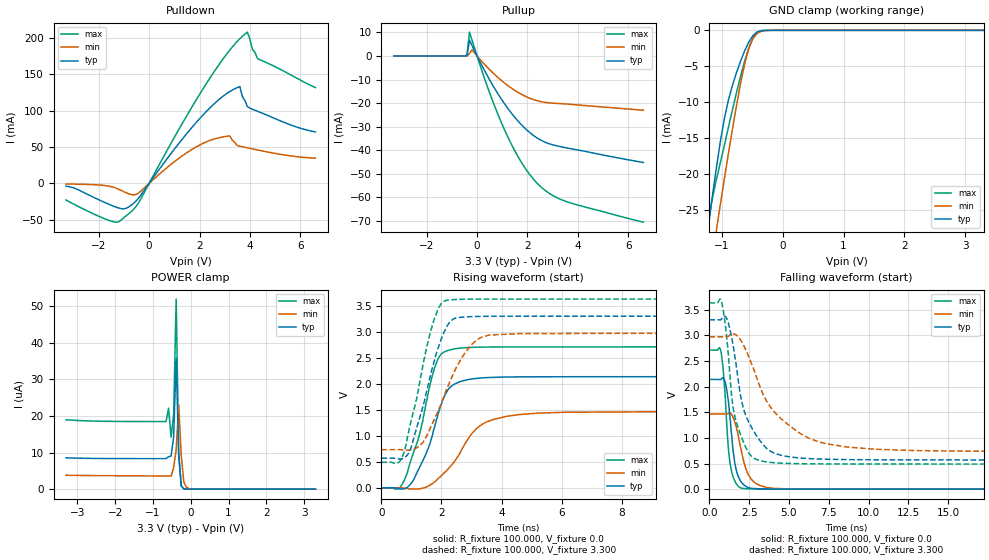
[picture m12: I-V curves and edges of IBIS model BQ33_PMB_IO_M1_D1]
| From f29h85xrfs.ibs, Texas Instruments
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|   Model BQ33_PMB_IO_M1_D1
[Model]   BQ33_PMB_IO_M1_D1
Model_type   I/O
Polarity   Non-Inverting
Enable   Active-Low
Vinl =   0.800V
Vinh =   1.350V
Vmeas =  1.650V
Cref =   100.000pF
Vref =   0.0V
|   typ   min   max
C_comp   1.646pF   1.624pF   1.798pF
[Model Spec]
Vinh   1.350V   1.350V   1.350V
Vinl   0.800V   0.800V   0.800V
[Temperature Range]   30   155   -40
[Voltage Range]   3.300V   2.970V   3.630V
[Pullup Reference]   3.300V   2.970V   3.630V
[Pulldown Reference]   0.0V   0.0V   0.0V
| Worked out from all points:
|   slope of the pulldown table from 0 to 0.495 V, typ, clamps not added: 20.8 ohm
|   slope of the pullup table from 0 to 0.495 V, typ, clamps not added: 49.3 ohm
|   GND clamp passes 1 mA (typ) near -0.51 V on its own axis
|   rising waveform, R_fixture 100.000, V_fixture 0.0: 20-80 % time 762ps typ, 1.14ns min, 712ps max; typ from 0 V to 2.14 V
|   rising waveform, R_fixture 100.000, V_fixture 3.300: 20-80 % time 773ps typ, 1.05ns min, 715ps max; typ from 0.57 V to 3.3 V
|   falling waveform, R_fixture 100.000, V_fixture 0.0: 20-80 % time 455ps typ, 712ps min, 376ps max; typ from 2.14 V to 0 V
|   falling waveform, R_fixture 100.000, V_fixture 3.300: 20-80 % time 1.3ns typ, 2.73ns min, 816ps max; typ from 3.3 V to 0.57 V
[Pulldown]
|Voltage   I(typ)   I(min)   I(max)
-3.3V     -3.922mA   -903.4uA   -22.93mA
-1.4V     -31.61mA   -5.56mA    -53.04mA
-700mV    -29.75mA   -15.51mA   -38.53mA
-400mV    -19.4mA    -12.71mA   -25.68mA
1.5V      68.79mA    42.37mA    93.49mA
2.8V      116.3mA    62.99mA    164.9mA
3.2V      126.4mA    65.38mA    183.5mA
3.6V      133.3mA    51.09mA    199.2mA
3.9V      105.6mA    48.92mA    208.3mA
4.1V      102mA      47.47mA    184.6mA
4.3V      99.3mA     46.01mA    171.8mA
6.6V      70.82mA    34.61mA    131.9mA
[Pullup]
|Voltage   I(typ)   I(min)   I(max)
-3.3V     -1.721nA   13.88nA    1.362nA
-500mV    17.31nA    18.01nA    59.06nA
-400mV    178uA      374.8nA    408.1uA
-300mV    6.695mA    1.073mA    10.14mA
-200mV    4.421mA    2.585mA    6.742mA
400mV     -8.225mA   -4.706mA   -12.71mA
1V        -18.86mA   -10.69mA   -29.15mA
1.7V      -28.49mA   -15.89mA   -44.05mA
2.3V      -34.18mA   -18.71mA   -53.02mA
2.8V      -37mA      -19.82mA   -57.81mA
3.5V      -38.88mA   -20.34mA   -61.59mA
6.6V      -45.18mA   -23.01mA   -70.51mA
[GND_clamp]
|Voltage   I(typ)   I(min)   I(max)
-3.3V     -172.4mA   -156.6mA   -199.3mA
-1.223V   -27.66mA   -35.43mA   -26.88mA
-1.156V   -23.42mA   -31.69mA   -23.55mA
-1.089V   -19.35mA   -27.98mA   -20.9mA
-1.022V   -15.58mA   -24.31mA   -18.47mA
-955mV    -12.3mA    -20.69mA   -16.02mA
-821mV    -7.634mA   -13.71mA   -11.02mA
-620mV    -2.823mA   -4.633mA   -4.248mA
-553mV    -1.627mA   -2.509mA   -2.447mA
-419mV    -233.9uA   -453.9uA   -290.2uA
-218mV    -985nA     -9.253uA   -449.5nA
3.3V      0A         0A         0A
[POWER_clamp]
|Voltage   I(typ)   I(min)   I(max)
-3.3V     8.55uA     3.797uA    18.96uA
-653mV    8.339uA    3.596uA    18.47uA
-586mV    8.872uA    3.591uA    22.11uA
-519mV    9.031uA    3.588uA    14.17uA
-452mV    14.26uA    5.833uA    20.33uA
-385mV    35.62uA    10.82uA    51.91uA
-318mV    9.151uA    22.94uA    10.03uA
-251mV    942nA      9.217uA    856.3nA
-184mV    84.85nA    2.059uA    62.73nA
-117mV    8.015nA    524.6nA    4.599nA
-50mV     1.476nA    168.6nA    663.4pA
3.3V      0A         0A         0A
[Ramp]
| variable   typ   min   max
dV/dt_r   1.282/0.762n   0.879/1.132n   1.626/0.713n
dV/dt_f   1.638/1.297n   1.342/2.726n   1.884/0.822n
R_load = 100.000
[Rising Waveform]
R_fixture= 100.000
V_fixture= 0.0
V_fixture_min= 0.0
V_fixture_max= 0.0
|time   V(typ)   V(min)   V(max)
0s        81.49uV    79.7uV     93.6uV
750ps     -21.09mV   -4.004mV   134.1mV
1.26ns    377.7mV    -19.52mV   1.008V
1.48ns    643.3mV    12.46mV    1.612V
1.94ns    1.509V     202.5mV    2.534V
2.24ns    1.904V     373mV      2.646V
2.87ns    2.079V     929.9mV    2.697V
3.68ns    2.124V     1.305V     2.708V
6.08ns    2.136V     1.453V     2.71V
100ns     2.137V     1.465V     2.71V
[Rising Waveform]
R_fixture= 100.000
V_fixture= 3.300
V_fixture_min= 2.970
V_fixture_max= 3.630
|time   V(typ)   V(min)   V(max)
0s        569.7mV    733.1mV    489.7mV
580ps     556.5mV    733.8mV    490.7mV
900ps     661.6mV    724.1mV    1.06V
1.36ns    1.524V     857.8mV    2.287V
1.77ns    2.469V     1.331V     3.268V
2.14ns    3.064V     1.852V     3.602V
2.47ns    3.264V     2.285V     3.622V
3.32ns    3.297V     2.893V     3.629V
4.59ns    3.3V       2.964V     3.63V
100ns     3.3V       2.97V      3.63V
[Falling Waveform]
R_fixture= 100.000
V_fixture= 0.0
V_fixture_min= 0.0
V_fixture_max= 0.0
|time   V(typ)   V(min)   V(max)
0s        2.137V     1.465V     2.71V
700ps     2.136V     1.465V     2.722V
960ps     2.116V     1.464V     1.981V
1.17ns    1.762V     1.471V     892.5mV
1.34ns    1.245V     1.478V     435mV
1.66ns    408.9mV    1.24V      120.9mV
2.17ns    83.53mV    526.4mV    12.75mV
2.93ns    10.43mV    109.8mV    3.77mV
5ns       1.747mV    6.738mV    830.6uV
100ns     275.2nV    4.142uV    154.1nV
[Falling Waveform]
R_fixture= 100.000
V_fixture= 3.300
V_fixture_min= 2.970
V_fixture_max= 3.630
|time   V(typ)   V(min)   V(max)
0s        3.3V       2.97V      3.63V
770ps     3.313V     2.97V      3.648V
1.09ns    3.326V     2.968V     2.96V
1.5ns     2.779V     3.027V     1.579V
2ns       1.767V     2.885V     1.028V
2.66ns    1.2V       2.433V     638.2mV
3.82ns    743.3mV    1.607V     521.9mV
6.82ns    588.3mV    927mV      492.6mV
12.92ns   570.6mV    752.1mV    489.9mV
100ns     569.6mV    733mV      489.6mV
